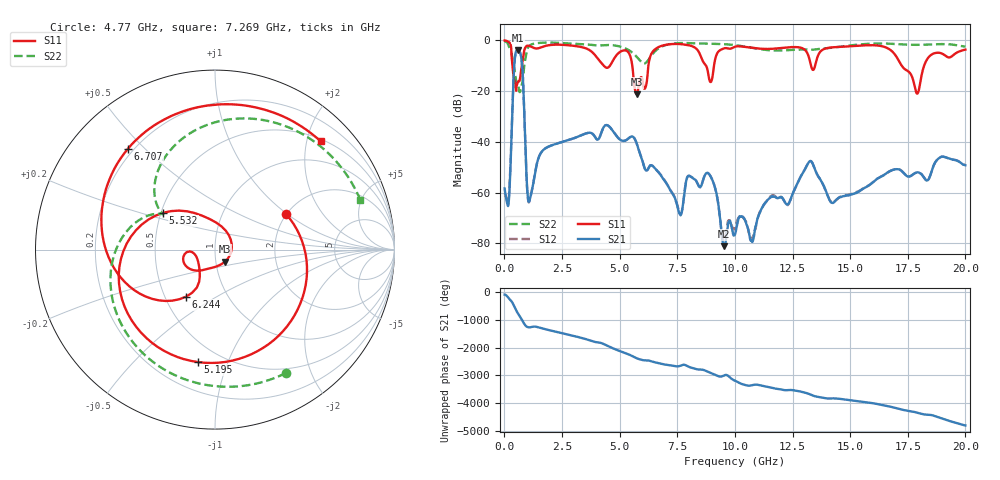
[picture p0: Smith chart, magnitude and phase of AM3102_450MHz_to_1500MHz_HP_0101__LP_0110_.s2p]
!Agilent Technologies,E8364B,MY43040894,A.07.50.67
!Agilent E8364B: A.07.50.67
!Date: Thursday, January 11, 2018 05:41:16
!Correction: S11(Full 2 Port(1,2))
!S21(Full 2 Port(1,2))
!S12(Full 2 Port(1,2))
!S22(Full 2 Port(1,2))
!S2P File: Measurements: S11, S21, S12, S22:
# Hz S  dB  R 50
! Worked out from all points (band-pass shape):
!   1601 points, 10 MHz to 20 GHz, reference 50 ohm
!   highest |S21| = -3.80 dB at 572.2 MHz (marker M1); lowest = -81.1 dB at 9.53 GHz (marker M2)
!   |S21| within 3 dB of the highest: 458.1 MHz to 731.7 MHz (273.7 MHz wide, 46 % of centre)
!   lowest |S11| = -21.2 dB at 5.745 GHz (marker M3), VSWR 1.19, Z = 55.4 - j7.43 ohm
!   |S11| at or under -10 dB: 349.3 MHz to 755.9 MHz (406.7 MHz wide, 73.6 % of centre); 5.548 GHz to 6.248 GHz (699.1 MHz wide, 11.9 % of centre); 17.24 GHz to 18.21 GHz (972.8 MHz wide, 5.49 % of centre)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
!   |S22| runs from -20.4 to -0.4 dB; largest |S21 - S12| = 0.0019
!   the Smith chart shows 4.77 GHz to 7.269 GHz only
!   S11 on the Smith chart (normalised r, x): 4.77 GHz: 2.00, +0.98; 5.195 GHz: 0.38, -0.79; 5.532 GHz: 0.51, +0.24; 6.244 GHz: 0.64, -0.37; 6.707 GHz: 0.18, +0.45; 7.269 GHz: 0.54, +2.27
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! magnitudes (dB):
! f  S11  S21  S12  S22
! 10 MHz  -0.1  -58.4  -60.1  -0.4
! 184.9 MHz  -0.6  -64.2  -62.8  -2.2
! 572.2 MHz  -16.6  -3.8  -3.8  -17.4
! 759.6 MHz  -9.8  -8.8  -8.8  -17.4
! 1.084 GHz  -2.2  -63.3  -63.4  -2.1
! 3.346 GHz  -2.7  -37.4  -37.4  -1.5
! 4.77 GHz  -7.1  -36.5  -36.5  -2.0
! 5.195 GHz  -4.0  -39.6  -39.6  -3.0
! 5.532 GHz  -9.0  -37.9  -37.9  -4.7
! 5.745 GHz  -21.2  -40.8  -40.8  -6.5
! 6.244 GHz  -10.2  -50.5  -50.5  -7.8
! 6.682 GHz  -2.7  -51.9  -52.0  -3.2
! 6.707 GHz  -2.6  -52.2  -52.2  -3.1
! 7.269 GHz  -1.5  -60.1  -60.1  -1.4
! 8.868 GHz  -14.5  -52.6  -52.6  -1.3
! 9.53 GHz  -3.2  -81.1  -78.7  -1.5
! 10.01 GHz  -2.5  -76.5  -73.8  -1.9
! 13.34 GHz  -11.1  -48.0  -48.0  -3.7
! 14.23 GHz  -2.8  -64.1  -63.8  -2.9
! 16.68 GHz  -3.4  -51.8  -51.9  -1.3
! 17.9 GHz  -21.0  -52.1  -52.1  -1.8
! 20 GHz  -3.7  -49.3  -49.1  -2.5
